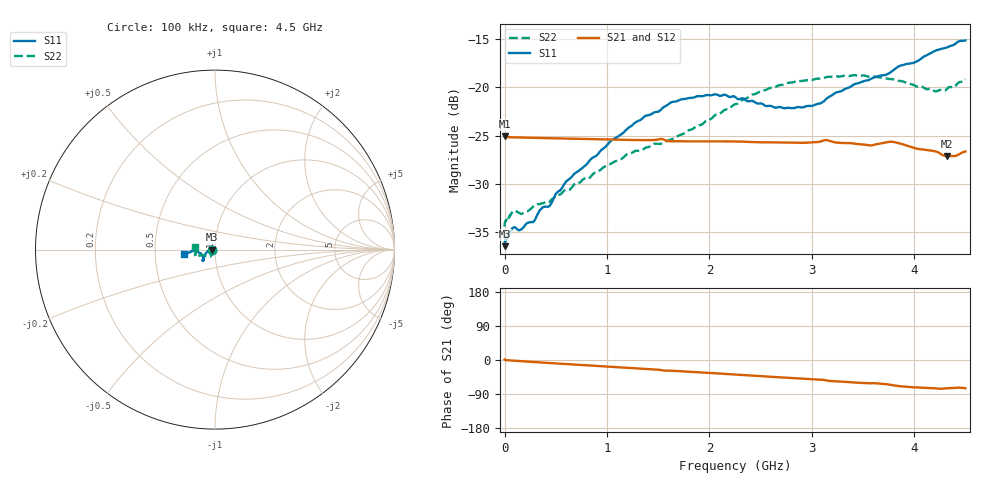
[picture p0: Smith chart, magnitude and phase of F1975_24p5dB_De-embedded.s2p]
! Integrated Device Technology
! Corporate Headquarters
! 6024 Silver Creek Valley Road
! San Jose, CA 95138  USA
! Phone:  1-408-284-8200
! Toll Free:  1-800-223-1366
! Webpage:  http://www.idt.com/
! Timing and RF Division
! 515 Groton Road, Suite 102
! Westford, MA 01886-6024
! Device:  F1975
! Description: 6-bit, 75 ohm, 0.5 dB Digital Step Attenuator
! Frequency:  5.0 MHz -  3.00 GHz
! Package:  4x4 mm QFN Plastic Package: 20 pin
! Ports:  2 RF, 11 DC
!  Pin  1  = D5 (16 dB)
!  Pin  2  = RF1  =  Port 1
!  Pin  3  = Serial Data In (DATA)
!  Pin  4  = Serial Clock (CLK)
!  Pin  5  = Serial Latch Enable (LE)
!  Pin  6  = VDD
!  Pin  7  = NC
!  Pin  8  = NC
!  Pin  9  = NC
!  Pin 10  = GND
!  Pin 11  = GND
!  Pin 12  = NC
!  Pin 13  = VMODE
!  Pin 14  = RF2  =  Port 2
!  Pin 15  = D4 (8 dB)
!  Pin 16  = D3 (4 dB)
!  Pin 17  = D2 (2 dB)
!  Pin 18  = NC
!  Pin 19  = D1 (1 dB)
!  Pin 20  = D0 (0.5 dB)
! State:  49
! Atten State:  24.5 dB
! Voltage:  +3.30 Volts
! Current:  0.560 mA
! Data:  The device was measured on a F1975 evaluation board which has
!  individual transmission lines to the RF pins.  Data was collected
!  using a calibrated network analyzer.  The evaluation board was
!  de-embedded using Automatic Fixture Removal (AFR).
!  The reference plane is the edge of the package pin.
! Misc:
!  Action Tracker AT0415
! Date Measured:  2018-02-08
! Date:  2018-03-26  MJV
! Note:
!  Integrated Device Technology supplies this data as a sample of measured
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# GHz S dB R 75
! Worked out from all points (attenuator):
!   291 points, 100 kHz to 4.5 GHz, reference 75 ohm
!   highest |S21| = -25.09 dB at 200 kHz (marker M1); lowest = -27.1 dB at 4.32 GHz (marker M2)
!   lowest |S11| = -36.4 dB at 100 kHz (marker M3), VSWR 1.03, Z = 72.8 - j0.00366 ohm
!   |S11| at or under -10 dB: start of sweep to end of sweep
!   |S22| runs from -34.4 to -18.8 dB; largest |S21 - S12| = 0.00016
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0.0001  -36.43 -179.9  -25.10 1.2  -25.10 1.2  -34.40 -179.2
0.0002  -36.33 -179.5  -25.09 1.2  -25.11 1.2  -34.35 -179.0
0.01  -35.85 -178.5  -25.16 -0.3  -25.16 -0.3  -33.80 -176.9
0.08  -34.52 -176.2  -25.18 -1.6  -25.18 -1.6  -32.82 -168.7
0.16  -34.70 -176.8  -25.20 -3.1  -25.20 -3.1  -33.09 -158.2
0.28  -33.94 -179.6  -25.23 -5.2  -25.23 -5.2  -32.32 -150.0
0.36  -32.53 -179.4  -25.25 -6.7  -25.25 -6.6  -32.00 -142.1
0.44  -32.28 -178.9  -25.27 -8.0  -25.27 -8.0  -31.85 -136.2
0.6  -29.75 -175.2  -25.32 -10.8  -25.31 -10.8  -30.59 -130.2
0.76  -28.34 -168.3  -25.35 -13.5  -25.35 -13.5  -29.57 -126.7
1.28  -23.63 -152.2  -25.46 -22.1  -25.46 -22.1  -26.56 -123.2
1.52  -22.40 -144.4  -25.36 -26.1  -25.36 -26.1  -25.86 -130.1
1.62  -21.60 -142.8  -25.60 -28.3  -25.59 -28.3  -25.42 -133.4
1.88  -20.94 -138.9  -25.59 -32.0  -25.59 -32.0  -23.98 -146.0
2.26  -21.08 -138.0  -25.61 -38.5  -25.61 -38.5  -21.74 -157.2
2.64  -22.12 -147.5  -25.70 -44.9  -25.70 -44.9  -20.00 -158.9
3.02  -21.87 -163.9  -25.68 -50.8  -25.68 -50.8  -19.20 -160.0
3.42  -19.68 -175.3  -25.84 -59.5  -25.83 -59.5  -18.75 -164.5
3.76  -18.53 -175.9  -25.64 -65.1  -25.63 -65.1  -19.16 -170.1
4.2  -16.26 -173.0  -26.62 -74.7  -26.61 -74.7  -20.42 178.3
4.32  -15.89 -172.7  -27.14 -74.7  -27.13 -74.6  -20.19 176.0
4.5  -15.17 -172.7  -26.64 -74.7  -26.64 -74.7  -19.15 173.5
